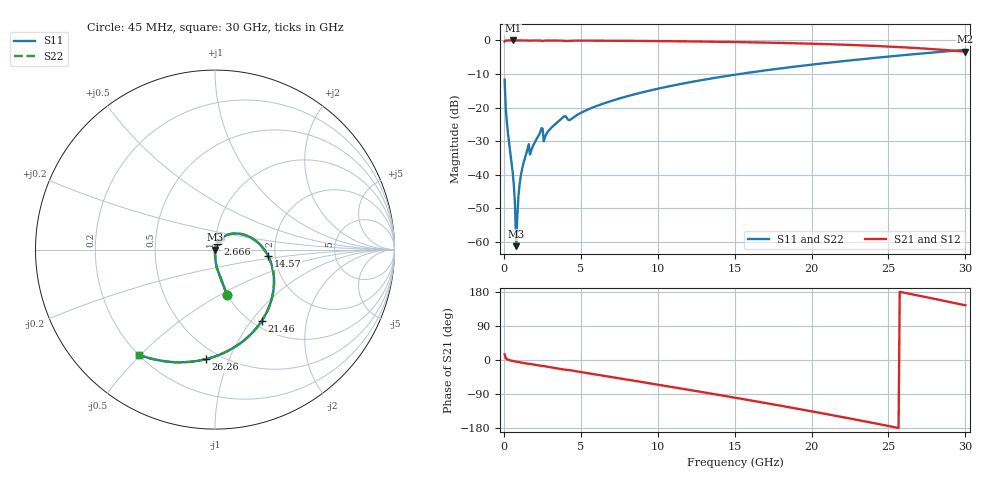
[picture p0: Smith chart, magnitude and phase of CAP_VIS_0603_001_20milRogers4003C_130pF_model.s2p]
! S-parameter model data by Modelithics Inc.  support@modelithics.com  813-866-6335  Tampa FL USA
! S-Parameter data specifications:
! Substrate: 20-mil Rogers 4003C, substrate thickness, H=0.508mm, Dielectric constant, Er=3.75
! PCB Mounting Pad Footprint: Pad width, PadW=0.90mm , Pad length, PadL=1.00mm , Pad gap, PadG (edge-to-edge)=1.00mm , Reference planes=3.0mm apart
! Created Wed Nov 18 13:32:00 2015
# hz S ma R 50
! 2 Port Network Data from SP1.SP block
! freq  magS11  angS11  magS21  angS21  magS12  angS12  magS22  angS22
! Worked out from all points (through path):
!   401 points, 45 MHz to 30 GHz, reference 50 ohm
!   highest |S21| = -0.01 dB at 569.2 MHz (marker M1); lowest = -3.3 dB at 30 GHz (marker M2)
!   group delay of S21, straight-line fit = 19.9 ps
!   lowest |S11| = -61.3 dB at 793.9 MHz (marker M3), VSWR 1.00, Z = 50.1 - j0.064 ohm
!   |S11| at or under -10 dB: start of sweep to 15.32 GHz
!   |S22| runs from -61.3 to -2.8 dB; largest |S21 - S12| = 0
!   S11 on the Smith chart (normalised r, x): 45 MHz: 1.00, -0.54; 2.666 GHz: 1.03, +0.07; 14.57 GHz: 1.83, -0.14; 21.46 GHz: 1.10, -1.13; 26.26 GHz: 0.42, -0.83; 30 GHz: 0.20, -0.49
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4.5e7  0.2612 -75.1  0.9651 14.9  0.9651 14.9  0.2612 -75.1
2.696625e8  0.04028 -88.6  0.9988 0.8  0.9988 0.8  0.04028 -88.6
5.692125e8  0.01092 -89.6  0.9994 -2.5  0.9994 -2.5  0.01092 -89.6
6.441e8  0.007032 -88.4  0.9994 -3.1  0.9994 -3.1  0.007032 -88.4
7.93875e8  0.0008648 -47.7  0.9993 -4.3  0.9993 -4.3  0.0008648 -47.7
9.4365e8  0.004788 76.4  0.9992 -5.4  0.9992 -5.4  0.004788 76.4
1.093425e9  0.009519 79.0  0.9991 -6.5  0.9991 -6.5  0.009519 79.0
1.467862e9  0.02128 77.1  0.9983 -9.2  0.9983 -9.2  0.02128 77.1
1.8423e9  0.02526 74.6  0.9977 -11.4  0.9977 -11.4  0.02526 74.6
2.366512e9  0.04355 70.6  0.9958 -15.3  0.9958 -15.3  0.04355 70.6
2.666062e9  0.03598 67.3  0.9953 -16.5  0.9953 -16.5  0.03598 67.3
3.864262e9  0.07241 59.3  0.9899 -25.0  0.9899 -25.0  0.07241 59.3
4.313588e9  0.06595 55.5  0.9889 -27.1  0.9889 -27.1  0.06595 55.5
5.062462e9  0.08488 56.1  0.9935 -32.2  0.9935 -32.2  0.08488 56.1
1.007992e10  0.1928 23.8  0.9781 -65.5  0.9781 -65.5  0.1928 23.8
1.457318e10  0.2979 -6.8  0.9505 -96.3  0.9505 -96.3  0.2979 -6.8
1.50225e10  0.3089 -10.0  0.9469 -99.5  0.9469 -99.5  0.3089 -10.0
2.003996e10  0.4371 -46.2  0.894 -135.7  0.894 -135.7  0.4371 -46.2
2.146282e10  0.4755 -56.9  0.8739 -146.4  0.8739 -146.4  0.4755 -56.9
2.505742e10  0.5769 -85.0  0.8098 -174.6  0.8098 -174.6  0.5769 -85.0
2.625562e10  0.6122 -94.7  0.7832 175.7  0.7832 175.7  0.6122 -94.7
3e10  0.7237 -126.1  0.6808 144.3  0.6808 144.3  0.7237 -126.1
